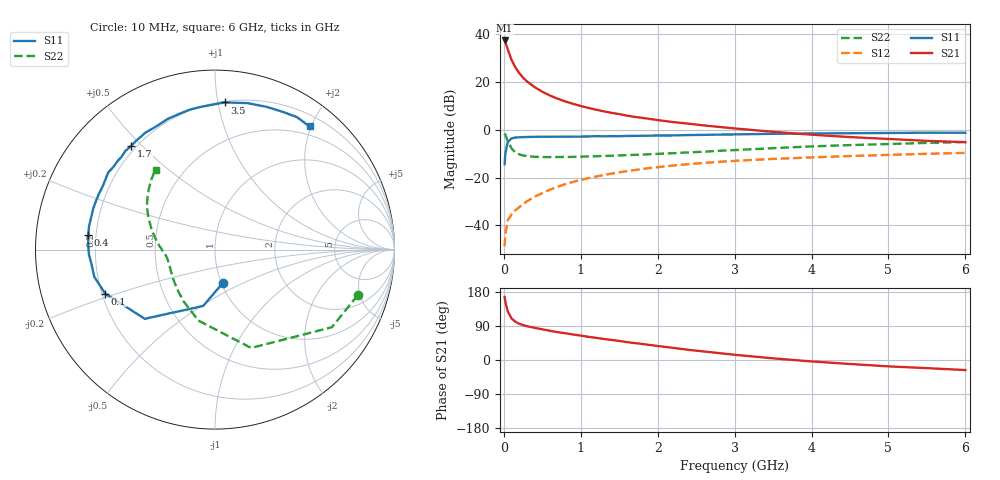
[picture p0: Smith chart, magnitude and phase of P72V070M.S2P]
! SIEMENS Small Signal Semiconductors
! BFP196
! Si NPN RF Bipolar Junction Transistor in SOT143
! VCE = 2 V  IC = 70 mA
! Common Emitter S-Parameters:  May  1996
# GHz  S  MA  R  50
!  f  S11  S21  S12  S22
! GHz  MAG  ANG  MAG  ANG  MAG  ANG  MAG  ANG
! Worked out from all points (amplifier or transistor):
!   36 points, 10 MHz to 6 GHz, reference 50 ohm
!   highest |S21| = 37.3 dB at 10 MHz (marker M1)
!   |S21| within 3 dB of that: start of sweep to 43.24 MHz
!   unconditionally stable (mu >= 1): 363.3 MHz to 4.85 GHz
!   at 250 MHz: K = 0.92, MSG = 26.4 dB, |S12| = -31.1 dB
!   at 1.4 GHz: K = 1.10, MAG = 10.8 dB, |S12| = -18.3 dB
!   at 6 GHz: K = 1.00, MSG = 2.2 dB, |S12| = -9.7 dB
!   S11 on the Smith chart (normalised r, x): 10 MHz: 1.02, -0.39; 100 MHz: 0.21, -0.18; 400 MHz: 0.17, +0.06; 1.7 GHz: 0.18, +0.47; 3.5 GHz: 0.21, +1.05; 6 GHz: 0.36, +1.97
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0.01  0.1908 -76.7  73.23 166.4  0.0037 76.1  0.8348 -17.7
0.02  0.321 -101.9  67.19 153.4  0.0066 68.2  0.7816 -33.6
0.05  0.5491 -135.4  48.08 128.5  0.0128 55.3  0.5838 -69.8
0.1  0.6593 -158.2  28.81 109.7  0.017 50.6  0.4062 -103.2
0.15  0.6893 -167.3  20.03 101.0  0.0208 52.7  0.3365 -121.6
0.2  0.6934 -173.5  15.27 95.7  0.0241 56.3  0.3058 -133.1
0.25  0.7029 -177.8  12.22 92.0  0.0278 58.8  0.2898 -141.6
0.3  0.7055 179.1  10.25 89.3  0.032 61.1  0.2813 -147.1
0.4  0.7111 173.4  7.758 84.8  0.0399 63.7  0.2725 -155.1
0.5  0.7139 169.3  6.209 81.0  0.0474 64.7  0.2685 -160.2
0.6  0.7129 165.1  5.172 77.1  0.0561 65.5  0.2682 -163.8
0.7  0.7158 161.3  4.445 73.4  0.0645 64.7  0.2689 -166.3
0.9  0.7172 154.7  3.473 67.3  0.0815 63.6  0.2711 -170.5
1.1  0.724 147.6  2.852 61.2  0.0974 61.5  0.2768 -173.4
1.3  0.7294 140.9  2.419 55.5  0.1137 58.8  0.2833 -176.0
1.7  0.7431 128.9  1.857 44.6  0.1437 53.3  0.2986 179.0
2.2  0.7606 115.4  1.446 32.1  0.1786 45.4  0.3233 172.8
2.8  0.792 100.3  1.144 18.2  0.2137 36.2  0.3634 164.0
3.5  0.8217 86.3  0.905 4.4  0.2458 26.2  0.4123 154.2
4.5  0.8455 70.3  0.702 -10.5  0.2824 14.0  0.4778 141.9
5.5  0.8681 58.2  0.586 -21.5  0.314 3.2  0.5305 131.7
6  0.8649 52.5  0.55 -26.5  0.3286 -2.6  0.5555 126.6
